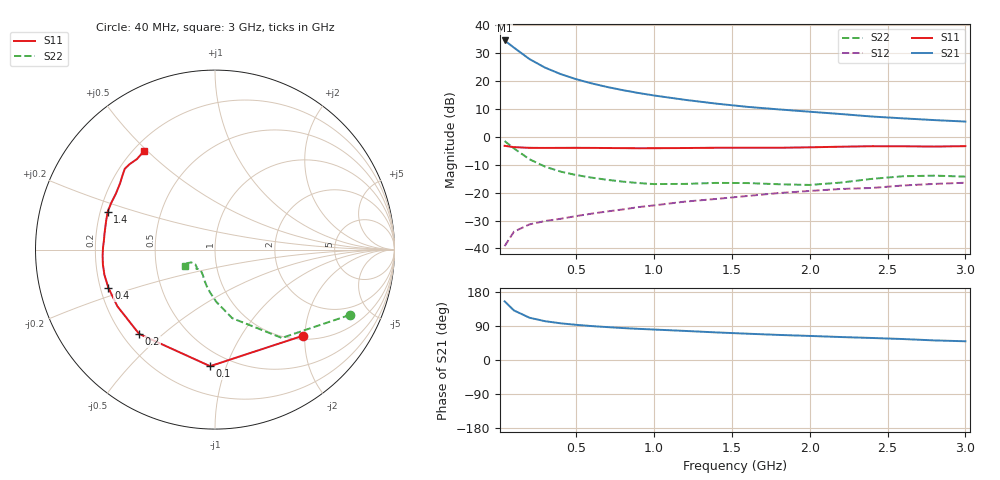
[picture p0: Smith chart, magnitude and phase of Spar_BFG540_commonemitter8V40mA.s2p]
! Filename:  BFG540K.S2P  Version:  3.0
! NXP part #: BFG540  Date: Feb 1992
! Bias condition: Vce=8V, Ic=40mA
! IN LINE PINNING: same data as with cross emitter pinning.
#  MHz  S  MA  R  50
! Freq  S11  S21  S12  S22  !GUM [dB]
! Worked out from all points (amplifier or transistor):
!   21 points, 40 MHz to 3 GHz, reference 50 ohm
!   highest |S21| = 34.4 dB at 40 MHz (marker M1)
!   |S21| within 3 dB of that: start of sweep to 110.5 MHz
!   unconditionally stable (mu >= 1): 749.2 MHz to end of sweep
!   at 300 MHz: K = 0.62, MSG = 27.4 dB, |S12| = -30.2 dB
!   at 1 GHz: K = 1.10, MAG = 17.7 dB, |S12| = -24.6 dB
!   at 3 GHz: K = 1.17, MAG = 8.5 dB, |S12| = -16.5 dB
!   lowest NFmin = 1.90 dB at 900 MHz
!   S11 on the Smith chart (normalised r, x): 40 MHz: 1.08, -1.97; 100 MHz: 0.39, -0.88; 200 MHz: 0.27, -0.42; 400 MHz: 0.23, -0.17; 1.4 GHz: 0.23, +0.16; 3 GHz: 0.24, +0.49
40  0.687 -44.2  52.66 154.8  0.011 69.5  0.834 -25.9
100  0.65 -92.4  39.17 130.8  0.02 53.2  0.617 -52.9
200  0.632 -132.0  24.43 111.5  0.027 45.1  0.394 -75.9
300  0.629 -149.9  17.18 102.4  0.031 45.1  0.291 -88.6
400  0.631 -160.2  13.17 96.8  0.034 48.1  0.237 -97.2
500  0.632 -167.2  10.67 92.8  0.038 50.7  0.206 -103.3
600  0.63 -172.5  8.971 89.5  0.042 53.6  0.185 -108.0
700  0.627 -177.0  7.733 86.8  0.046 55.8  0.169 -111.9
800  0.624 179.0  6.793 84.3  0.05 57.6  0.157 -115.6
900  0.621 175.3  6.051 82.2  0.055 59.2  0.148 -119.7
1000  0.622 171.6  5.458 80.4  0.059 60.9  0.142 -123.8
1200  0.627 165.4  4.559 76.7  0.069 62.8  0.143 -130.7
1400  0.634 160.5  3.902 72.8  0.077 63.5  0.149 -133.5
1600  0.634 155.9  3.417 69.4  0.087 65.1  0.148 -134.0
1800  0.634 150.7  3.078 66.2  0.098 64.7  0.141 -136.2
2000  0.645 145.1  2.796 63.5  0.107 65.4  0.137 -143.6
2200  0.662 141.0  2.542 60.6  0.116 65.2  0.151 -151.9
2400  0.675 138.1  2.293 58.1  0.121 65.6  0.176 -154.3
2600  0.673 135.0  2.127 55.3  0.134 64.6  0.196 -152.1
2800  0.666 130.8  1.981 51.7  0.143 62.3  0.201 -149.2
3000  0.677 125.7  1.864 49.4  0.15 62.8  0.193 -150.8
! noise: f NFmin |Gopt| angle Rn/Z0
900  1.9  0.263  155  0.14
2000  2.6  0.494  -162  0.13
